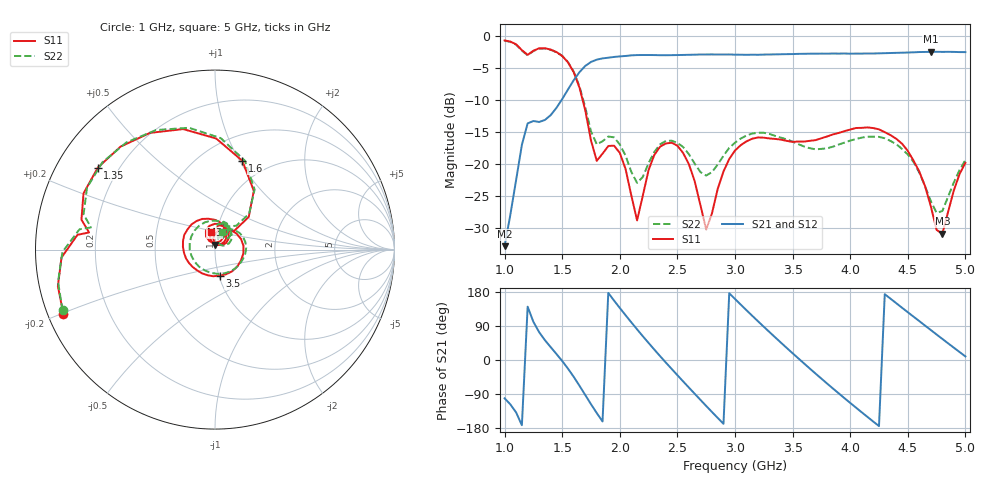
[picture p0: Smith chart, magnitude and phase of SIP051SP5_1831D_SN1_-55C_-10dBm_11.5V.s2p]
# GHz  S  dB  R  50
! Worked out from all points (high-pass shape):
!   81 points, 1 GHz to 5 GHz, reference 50 ohm
!   highest |S21| = -2.52 dB at 4.7 GHz (marker M1); lowest = -32.9 dB at 1 GHz (marker M2)
!   |S21| within 3 dB of the highest: 1.659 GHz to end of sweep
!   lowest |S11| = -31.0 dB at 4.8 GHz (marker M3), VSWR 1.06, Z = 49.7 + j2.8 ohm
!   |S11| at or under -10 dB: 1.677 GHz to end of sweep
!   |S22| runs from -27.7 to -0.8 dB; largest |S21 - S12| = 0.0019
!   S11 on the Smith chart (normalised r, x): 1 GHz: 0.04, -0.20; 1.35 GHz: 0.12, +0.31; 1.6 GHz: 0.76, +1.03; 3.5 GHz: 1.01, -0.30; 5 GHz: 0.94, +0.19
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1  -0.75 -157.1  -32.91 -101.1  -32.94 -101.1  -0.78 -158.3
1.2  -3.00 172.3  -13.71 140.8  -13.72 140.9  -3.07 169.9
1.35  -1.97 145.0  -13.18 52.3  -13.17 52.3  -2.01 142.2
1.5  -3.17 104.8  -9.92 -2.7  -9.91 -2.7  -3.17 102.0
1.6  -5.72 72.9  -6.96 -44.5  -6.97 -44.5  -5.63 71.5
1.7  -11.65 44.1  -4.74 -92.3  -4.73 -92.3  -11.19 46.4
1.8  -19.57 68.9  -3.75 -140.0  -3.76 -140.0  -16.99 64.4
1.95  -17.20 73.3  -3.33 156.8  -3.34 156.8  -15.89 65.4
2.15  -28.88 92.1  -3.04 80.9  -3.04 80.9  -23.01 70.5
2.35  -17.35 103.8  -3.06 10.1  -3.04 10.1  -16.98 84.0
2.5  -17.20 64.2  -3.03 -40.0  -3.03 -40.1  -16.75 55.9
2.65  -22.75 30.9  -2.98 -89.1  -2.97 -89.0  -20.00 40.7
2.75  -30.32 60.0  -2.94 -121.3  -2.93 -121.2  -21.86 53.2
3  -17.96 65.8  -2.97 161.0  -2.97 161.0  -16.74 51.4
3.25  -15.95 -7.1  -2.96 87.7  -2.96 87.8  -15.18 3.6
3.5  -16.61 -80.2  -2.88 17.8  -2.88 17.8  -16.57 -55.7
3.7  -16.33 -130.7  -2.82 -36.0  -2.81 -36.0  -17.77 -115.7
4  -14.68 164.9  -2.81 -113.2  -2.81 -113.2  -16.40 150.5
4.35  -15.55 91.4  -2.71 161.7  -2.73 161.7  -16.46 66.2
4.7  -26.69 42.5  -2.52 79.0  -2.53 79.0  -25.86 25.6
4.8  -30.97 95.0  -2.54 55.6  -2.54 55.6  -27.42 59.9
5  -19.90 102.6  -2.58 9.5  -2.58 9.5  -19.45 67.6
